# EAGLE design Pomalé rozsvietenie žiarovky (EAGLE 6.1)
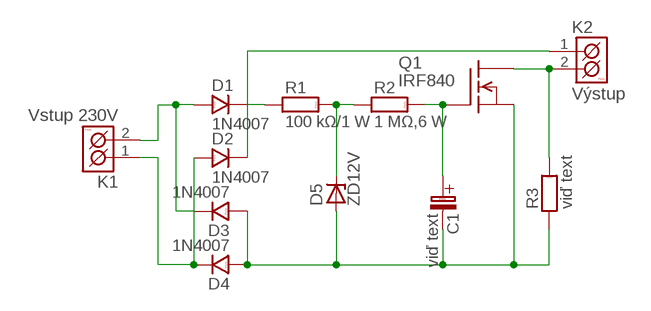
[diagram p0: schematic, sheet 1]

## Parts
C1  viď text  C-ELEKTROLYT_2,5  [C-EL_2,5]
D1  1N4007  1N4007_10  [DO41]
D2  1N4007  1N4007_10  [DO41]
D3  1N4007  1N4007_10  [DO41]
D4  1N4007  1N4007_10  [DO41]
D5  ZD12V  BZX85  [DO41Z10]
K1  Vstup 230V  ARK500/2  [ARK500/2]
K2  Výstup  ARK500/2  [ARK500/2]
Q1  IRF840  [TO220]
R1  100 kΩ/1 W  R__2W  [R-_2W]
R2  1 MΩ,6 W  R_10  [R-10]
R3  viď text  R__5W  [R-_5W]

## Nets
N$1: D1.A D3.K K1.2(K2)
N$2: D2.A D4.K K1.1(K1)
N$3: D1.K D2.K K2.1(K1) R1.1
N$4: C1.C-(C_EL-) D3.A D4.A D5.A Q1.3(S) R3.1
N$5: C1.C+(C_EL+) Q1.1(G) R2.2
N$6: D5.C R1.2 R2.1
N$7: K2.2(K2) Q1.2(D) R3.2

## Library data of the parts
C1 = #PaJa_30:C-ELEKTROLYT: Kondenzator - elektrolyticky
D1-D4 = #PaJa_30:1N4007: Usmernovaci dioda - 1A, 1000V
D5 = diode:BZX85: Z DIODE
K1 K2 = #PaJa_konektory:ARK500/2: Svorkovnice - roztec 5mm - dvojita
Q1 = transistor-fet:IRF840: N-Channel Enhancement MOSFET (HEXFET); 500V; 8A; 0,85Ohm
R1-R3 = #PaJa_30:R: Rezistor

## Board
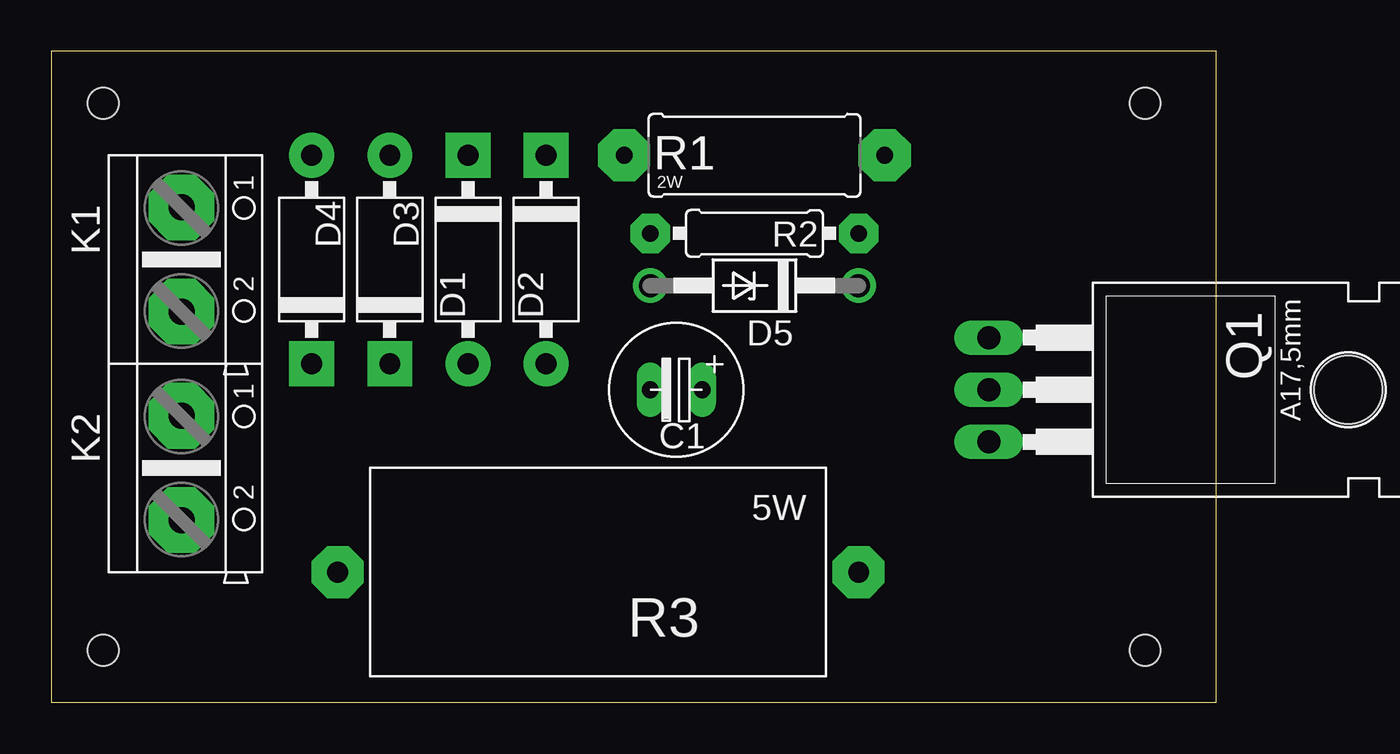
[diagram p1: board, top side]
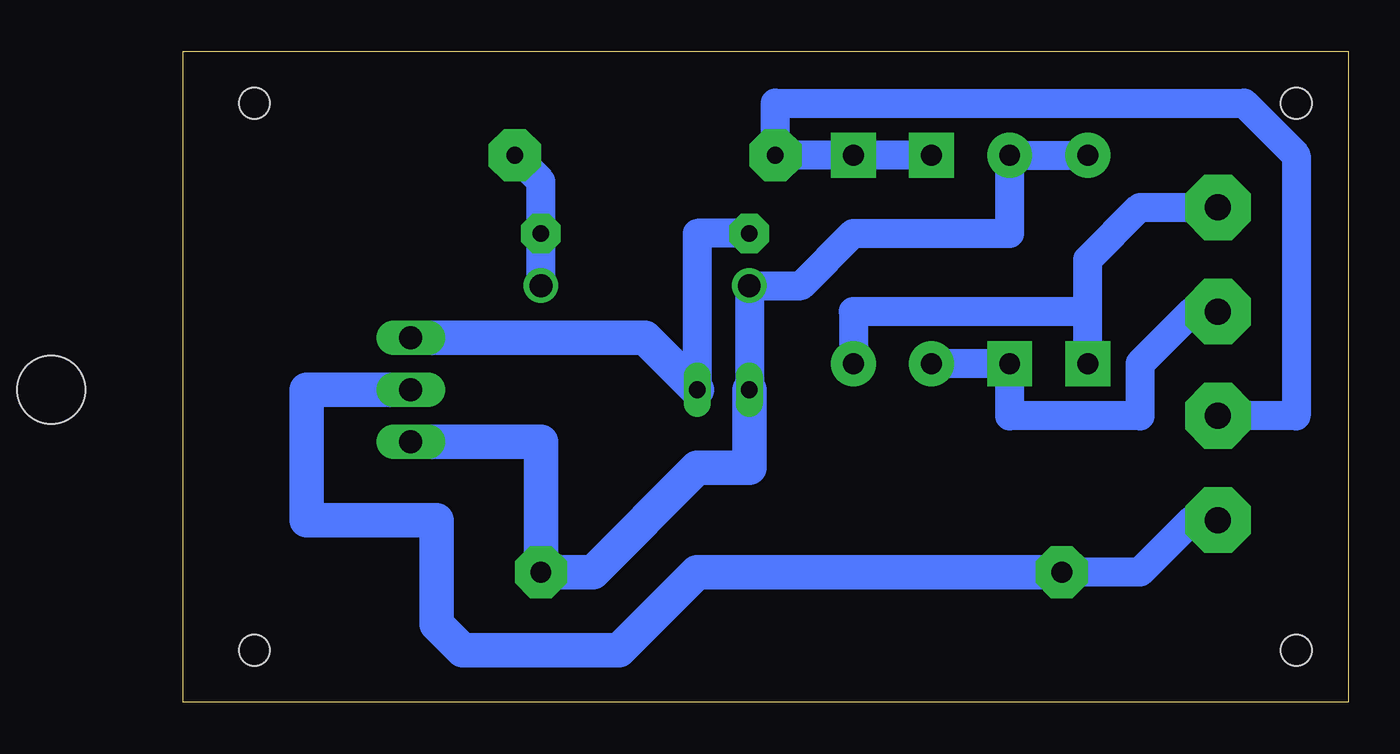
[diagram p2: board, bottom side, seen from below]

Size 56.82 x 31.74 mm. Coordinates in mm from the lower left corner, seen from the top.
Outline: 0,0 56.82,0 56.82,31.74 0,31.74 0,0
Copper layers (1*16): Top 0.035mm / dielectric 1.5mm / Bottom 0.035mm
Design rules: minimum track width 10mil, minimum drill 24mil, track to track 8mil, track to pad 8mil, pad to pad 8mil, via to via 8mil, smd to smd 8mil, copper to edge 40mil, drill to drill 8mil, minimum pad ring 10mil, minimum via ring 8mil, stop-mask expansion 4mil, vias tented up to drill 0mil, thermal gap 10mil
Holes 1.5 mm at 2.54,2.54 53.34,2.54 53.34,29.21 2.54,29.21

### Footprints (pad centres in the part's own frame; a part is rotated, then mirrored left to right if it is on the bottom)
C-EL_2,5 = drill 0.813 pad 1.27 long: C+ -1.27,0; C- 1.27,0
DO41 = drill 1.016 pad 2.184: A -5.08,0 | drill 1.016 pad 2.184 square: K 5.08,0
DO41Z10 = drill 1.118: A 5.08,0; C -5.08,0
ARK500/2 = drill 1.27 pad 3.2 octagon: 1 -2.54,0; 2 2.54,0
TO220 = drill 1.118 long: 1 -2.54,-6.35; 2 0,-6.35; 3 2.54,-6.35 | hole 3.302: 0,11.176
R-_2W = drill 0.813 pad 2.54 octagon: 1 -6.35,0; 2 6.35,0
R-10 = drill 0.813 pad 1.93 octagon: 1 -5.08,0; 2 5.08,0
R-_5W = drill 1.016 pad 2.54 octagon: 1 -12.7,0; 2 12.7,0

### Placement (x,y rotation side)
C1  30.48,15.24 180 top
D1  20.32,21.59 90 top
D2  24.13,21.59 90 top
D3  16.51,21.59 270 top
D4  12.7,21.59 270 top
D5  34.29,20.32 180 top
K1  6.35,21.59 270 top
K2  6.35,11.43 270 top
Q1  52.07,15.24 270 top
R1  34.29,26.67 0 top
R2  34.29,22.86 180 top
R3  26.67,6.35 180 top

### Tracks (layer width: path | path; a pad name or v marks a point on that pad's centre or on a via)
N$1
  Bottom 1.422: K1.2 7.62,19.05 10.16,16.51 10.16,13.97 16.51,13.97 D3.K D1.A
N$2
  Bottom 1.422: 12.7,19.05 24.13,19.05 D2.A | D4.K 12.7,19.05 | 12.7,19.05 12.7,21.59 10.16,24.13 K1.1
N$3
  Bottom 1.422: D1.K D2.K R1.1 27.94,29.21 5.08,29.21 2.54,26.67 2.54,13.97 K2.1
N$4
  Bottom 1.422: D4.A D3.A 16.51,22.86 24.13,22.86 26.67,20.32 D5.A C1.C-
  Bottom 1.676: 44.45,12.7 Q1.3 39.37,12.7 R3.1 36.83,6.35 31.75,11.43 29.21,11.43 C1.C-
N$5
  Bottom 1.422: R2.2 31.75,22.86 C1.C+
  Bottom 1.676: Q1.1 34.29,17.78 C1.C+
N$6
  Bottom 1.422: R1.2 39.37,25.4 R2.1 D5.C
N$7
  Bottom 1.422: K2.2 7.62,8.89 10.16,6.35 R3.2
  Bottom 1.676: Q1.2 50.8,15.24 50.8,8.89 44.45,8.89 44.45,3.81 43.18,2.54 35.56,2.54 31.75,6.35 R3.2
